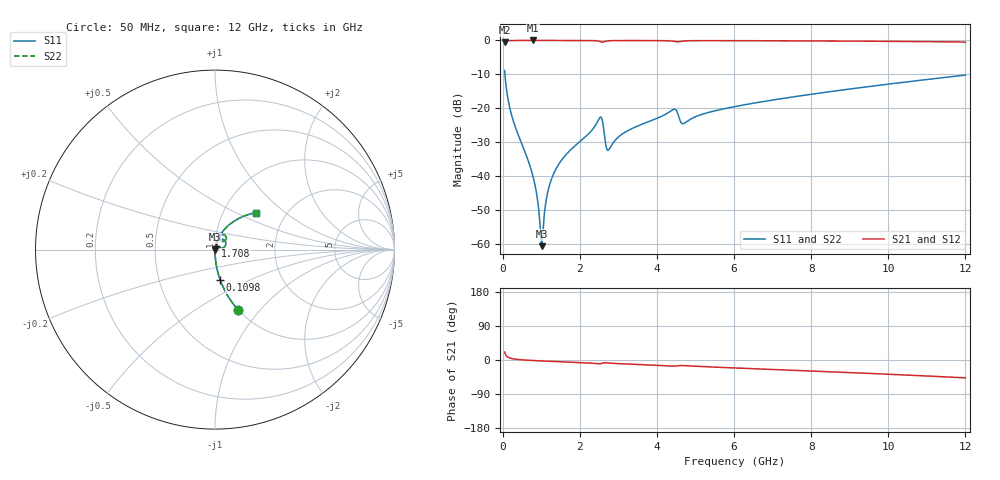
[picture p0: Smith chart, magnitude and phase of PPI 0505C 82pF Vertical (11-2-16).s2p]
# GHz S MA R 50
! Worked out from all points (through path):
!   1601 points, 50 MHz to 12 GHz, reference 50 ohm
!   highest |S21| = -0.01 dB at 774.5 MHz (marker M1); lowest = -0.6 dB at 50 MHz (marker M2)
!   group delay of S21, straight-line fit = 11.2 ps
!   lowest |S11| = -60.7 dB at 1.013 GHz (marker M3), VSWR 1.00, Z = 50.1 + j0.0045 ohm
!   |S11| at or under -10 dB: 57.84 MHz to end of sweep
!   |S22| runs from -60.7 to -8.9 dB; largest |S21 - S12| = 0
!   S11 on the Smith chart (normalised r, x): 50 MHz: 1.00, -0.77; 109.8 MHz: 1.00, -0.35; 1.708 GHz: 1.01, +0.05; 12 GHz: 1.42, +0.65
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0.05  0.3599 -69.0  0.9327 21.0  0.9327 21.0  0.3599 -69.0
0.10975  0.1715 -80.3  0.9848 9.6  0.9848 9.6  0.1715 -80.3
0.2740625  0.0653 -86.5  0.9973 3.1  0.9973 3.1  0.0653 -86.5
0.7744688  0.01046 -86.9  0.9991 -1.3  0.9991 -1.3  0.01046 -86.9
0.8715625  0.005847 -83.4  0.9991 -1.8  0.9991 -1.8  0.005847 -83.4
0.9686562  0.0019 -64.1  0.999 -2.3  0.999 -2.3  0.0019 -64.1
1.013469  0.0009219 2.8  0.999 -2.5  0.999 -2.5  0.0009219 2.8
1.147906  0.005081 75.8  0.9989 -3.1  0.9989 -3.1  0.005081 75.8
1.252469  0.008571 79.5  0.9989 -3.6  0.9989 -3.6  0.008571 79.5
1.708063  0.02263 81.1  0.9983 -5.5  0.9983 -5.5  0.02263 81.1
2.044156  0.03376 79.7  0.9974 -7.0  0.9974 -7.0  0.03376 79.7
2.529625  0.07347 48.9  0.9598 -9.9  0.9598 -9.9  0.07347 48.9
2.693938  0.02565 28.6  0.979 -7.6  0.979 -7.6  0.02565 28.6
2.753687  0.02447 52.0  0.9874 -8.1  0.9874 -8.1  0.02447 52.0
3.149531  0.04339 75.4  0.9956 -10.3  0.9956 -10.3  0.04339 75.4
4.038312  0.0724 72.8  0.9933 -14.2  0.9933 -14.2  0.0724 72.8
4.456563  0.09688 55.3  0.9649 -16.3  0.9649 -16.3  0.09688 55.3
4.695563  0.05956 58.2  0.9808 -14.9  0.9808 -14.9  0.05956 58.2
6.025  0.1058 67.5  0.9912 -21.0  0.9912 -21.0  0.1058 67.5
8.019156  0.1611 60.0  0.9835 -29.0  0.9835 -29.0  0.1611 60.0
10.01331  0.227 51.5  0.9698 -37.6  0.9698 -37.6  0.227 51.5
12  0.3078 42.1  0.9465 -47.1  0.9465 -47.1  0.3078 42.1
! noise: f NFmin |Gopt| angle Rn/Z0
0.05  0.0003751  0.8598  0.3776  0.0005728
1.372  0.003901  0.6681  3.358  0.002255
2.701  0.02286  0.8747  6.707  0.03926
4.031  0.01244  0.6907  9.71  0.007771
5.36  0.0137  0.6388  12.75  0.007074
6.682  0.01398  0.5765  15.37  0.005892
8.012  0.0159  0.56  18.07  0.006343
9.341  0.01817  0.5545  20.74  0.007083
10.67  0.02072  0.5556  23.36  0.008034
12  0.02359  0.5618  25.96  0.009229
